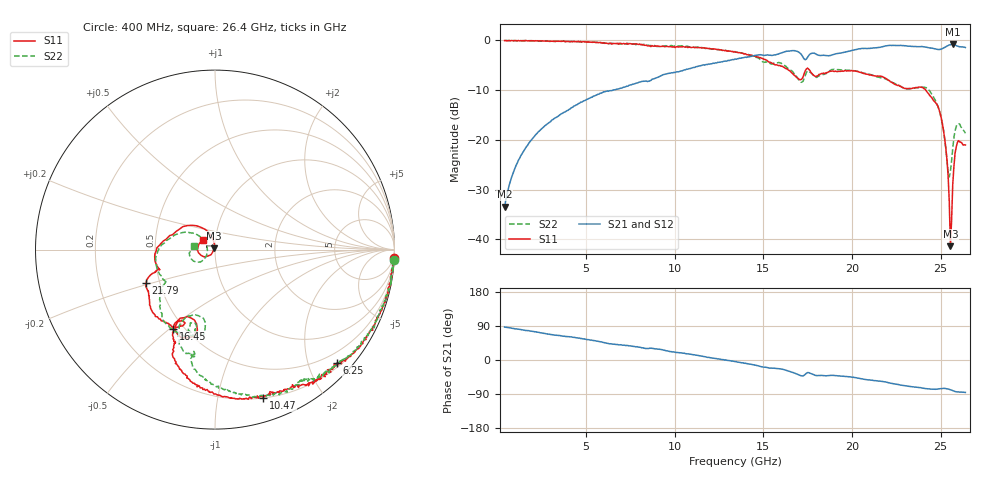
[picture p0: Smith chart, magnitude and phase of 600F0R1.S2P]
!  American Technical Ceramics  Date:  11/23/05
!  One Norden Lane
!  Huntington Station,  NY.  11746-2102
!  Tel:  (631) 622-4700  Fax:  (631) 622-4748
!  Part Number  600F0R1  Mounting Orientation: Horizontal
!  Description: Ultra Low ESR Microwave capacitors
!  Application: Coupling, Bypass, Tuning, DC Block
!  Filters, Matching
# GHZ S DB R 50
! Freq  |S11|  S11 Ph  |S21|  S21 Ph  |S12|  S12 Ph  |S22|  S22 Ph
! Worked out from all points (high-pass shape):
!   401 points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, 400 MHz to 26.4 GHz, reference 50 ohm
!   highest |S21| = -0.78 dB at 25.68 GHz (marker M1); lowest = -33.5 dB at 400 MHz (marker M2)
!   |S21| within 3 dB of the highest: 13.47 GHz to 17.32 GHz (3.852 GHz wide, 25 % of centre); 17.41 GHz to end of sweep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
!   lowest |S11| = -41.4 dB at 25.55 GHz (marker M3), VSWR 1.02, Z = 49.4 + j0.641 ohm
!   |S11| at or under -10 dB: 24.17 GHz to end of sweep
!   |S22| runs from -27.5 to 0.0 dB; largest |S21 - S12| = 0.0098
!   S11 on the Smith chart (normalised r, x): 400 MHz: 2, -40; 6.25 GHz: 0.28, -2.52; 10.47 GHz: 0.20, -1.36; 16.45 GHz: 0.44, -0.51; 21.79 GHz: 0.42, -0.19; 26.4 GHz: 0.86, +0.10
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0.4  -0.02 -2.8  -33.45 86.9  -33.48 86.7  0.00 -3.3
1.05  -0.03 -7.2  -25.12 82.1  -25.13 81.3  -0.05 -9.1
1.895  -0.05 -13.7  -20.07 76.2  -20.06 76.4  -0.04 -14.0
4.755  -0.31 -33.9  -12.38 56.6  -12.42 56.1  -0.33 -32.1
6.25  -0.65 -42.8  -10.22 43.5  -10.19 43.4  -0.60 -41.8
9.11  -1.16 -62.9  -7.31 28.8  -7.32 28.8  -1.23 -56.8
10.475  -1.22 -72.0  -6.01 17.9  -6.00 18.6  -1.24 -66.8
13.4  -2.26 -97.5  -3.72 -4.3  -3.73 -4.4  -2.24 -88.5
16.455  -6.04 -117.8  -2.14 -29.7  -2.14 -29.7  -5.71 -113.0
17.235  -7.39 -103.9  -3.36 -42.1  -3.39 -41.7  -8.21 -99.5
17.755  -6.73 -117.3  -2.57 -37.0  -2.59 -36.9  -6.73 -108.6
21.785  -7.41 -154.1  -1.21 -57.3  -1.20 -57.0  -7.60 -137.7
22.11  -8.08 -157.9  -1.00 -60.1  -0.96 -59.9  -8.10 -141.1
24.19  -10.13 175.8  -1.36 -75.6  -1.31 -75.7  -9.50 -171.3
24.84  -13.15 144.4  -1.81 -76.8  -1.78 -76.9  -13.16 155.9
25.23  -19.72 110.6  -1.41 -74.9  -1.38 -74.9  -19.79 138.3
25.425  -27.21 98.5  -1.01 -76.5  -0.99 -76.4  -26.40 159.6
25.555  -41.38 130.5  -0.87 -78.5  -0.83 -78.7  -26.34 -155.9
25.685  -29.07 -127.7  -0.78 -80.8  -0.75 -81.1  -21.78 -138.4
25.815  -22.76 -146.2  -0.87 -83.2  -0.87 -83.3  -18.21 -144.9
25.945  -20.55 -169.5  -1.13 -84.3  -1.12 -84.2  -16.83 -160.0
26.4  -21.02 141.4  -1.42 -85.5  -1.40 -85.5  -18.67 169.4
